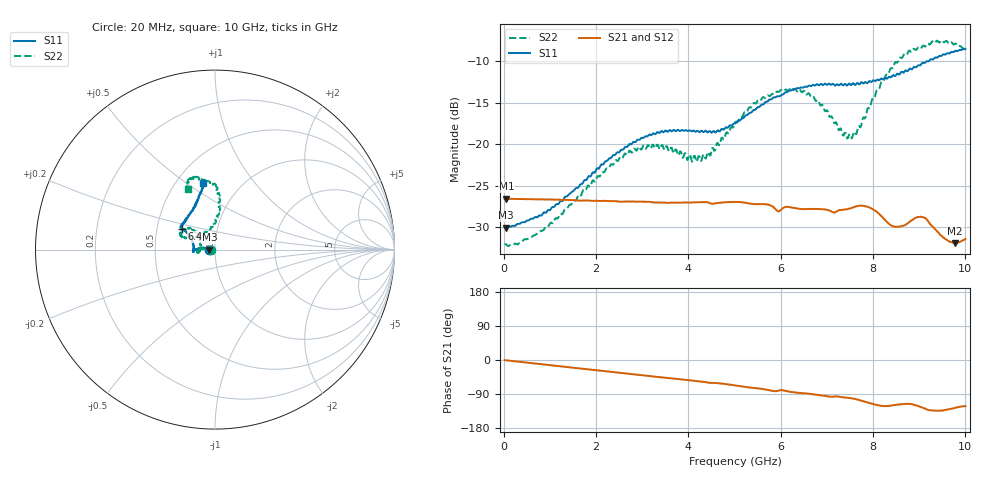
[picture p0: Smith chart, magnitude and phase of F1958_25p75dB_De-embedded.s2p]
! Integrated Device Technology
! Corporate Headquarters
! 6024 Silver Creek Valley Road
! San Jose, CA 95138  USA
! Phone:  1-408-284-8200
! Toll Free:  1-800-223-1366
! Webpage:  http://www.idt.com/
! Timing and RF Division
! 515 Groton Road, Suite 102
! Westford, MA 01886-6024
! Device:  F1958
! Description: 7-bit 0.25 dB Digital Step Attenuator
! Frequency:  0.001 -  6.000 GHz
! Package:  4x4 mm Thin QFN Plastic Package: 24 pin
! Ports:  2 RF, 12 DC
!  Pin  1  = D0
!  Pin  2  = VDD
!  Pin  3  = VMODE
!  Pin  4  = GND
!  Pin  5  = RF1  =  Port 1
!  Pin  6  = GND
!  Pin  7  = GND
!  Pin  8  = GND
!  Pin  9  = GND
!  Pin 10  = GND
!  Pin 11  = GND
!  Pin 12  = GND
!  Pin 13  = GND
!  Pin 14  = RF2  =  Port 2
!  Pin 15  = GND
!  Pin 16  = LE
!  Pin 17  = CLK
!  Pin 18  = DATA
!  Pin 19  = D6
!  Pin 20  = D5
!  Pin 21  = D4
!  Pin 22  = D3
!  Pin 23  = D2
!  Pin 24  = D1
! State:  103
! Atten State:  25.75 dB
! Voltage:  +3.30 Volts
! Current:  0.258 mA
! Data:  The device was measured on a F1958 evaluation board which has
!  individual transmission lines to the RF pins.  Data was collected
!  using a calibrated network analyzer.  The evaluation board was
!  de-embedded using Automatic Fixture Removal (AFR).
!  The reference plane is the edge of the package pin.
! Misc:
!  Action Tracker AT0419
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# GHz S dB R 50
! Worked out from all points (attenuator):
!   500 points, 20 MHz to 10 GHz, reference 50 ohm
!   highest |S21| = -26.60 dB at 60 MHz (marker M1); lowest = -32.0 dB at 9.78 GHz (marker M2)
!   lowest |S11| = -30.1 dB at 40 MHz (marker M3), VSWR 1.06, Z = 47 - j0.0406 ohm
!   |S11| at or under -10 dB: start of sweep to 9.153 GHz
!   |S22| runs from -32.3 to -7.5 dB; largest |S21 - S12| = 0.00032
!   S11 on the Smith chart (normalised r, x): 20 MHz: 0.94, -0.00; 6.4 GHz: 0.67, +0.16; 10 GHz: 0.68, +0.58
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0.02  -30.07 -178.9  -26.61 -0.3  -26.61 -0.3  -32.10 -178.9
0.04  -30.10 -179.2  -26.61 -0.5  -26.60 -0.5  -32.08 -178.3
0.06  -30.07 180.0  -26.60 -0.8  -26.59 -0.8  -32.14 -178.3
0.84  -28.47 170.9  -26.67 -11.6  -26.66 -11.6  -30.45 172.8
1.7  -24.80 170.8  -26.81 -22.9  -26.81 -22.9  -25.82 171.8
2.62  -20.39 176.9  -26.93 -35.1  -26.91 -35.1  -21.14 -179.3
3.36  -18.62 -175.9  -27.05 -45.1  -27.06 -45.3  -20.40 -169.4
4.24  -18.55 -179.2  -27.02 -56.3  -27.03 -56.4  -21.48 168.9
4.5  -18.61 174.9  -27.19 -60.4  -27.20 -60.5  -20.85 151.6
5.02  -17.48 160.5  -26.97 -67.3  -26.98 -67.2  -17.31 138.4
5.6  -15.20 150.6  -27.25 -76.3  -27.27 -76.3  -14.39 140.2
5.94  -14.19 148.2  -28.09 -81.5  -28.11 -81.4  -13.66 148.6
6.4  -13.25 147.7  -27.81 -86.8  -27.83 -86.7  -13.37 155.6
6.68  -12.89 146.6  -27.83 -90.0  -27.84 -90.0  -14.29 157.5
7.5  -12.72 138.3  -27.77 -100.4  -27.77 -100.2  -18.79 119.8
7.68  -12.68 135.4  -27.45 -104.9  -27.45 -104.8  -17.85 100.0
7.9  -12.48 129.0  -27.60 -112.8  -27.59 -112.9  -15.59 89.6
8.34  -11.86 119.1  -29.60 -121.4  -29.60 -121.4  -11.42 84.1
8.66  -11.37 113.4  -29.85 -116.1  -29.85 -116.3  -9.23 87.7
9.08  -10.15 107.3  -28.80 -125.9  -28.85 -126.1  -8.08 98.7
9.78  -8.71 100.4  -31.95 -126.3  -32.00 -126.6  -7.84 111.5
10  -8.50 100.0  -31.44 -121.7  -31.50 -121.5  -8.61 113.5
